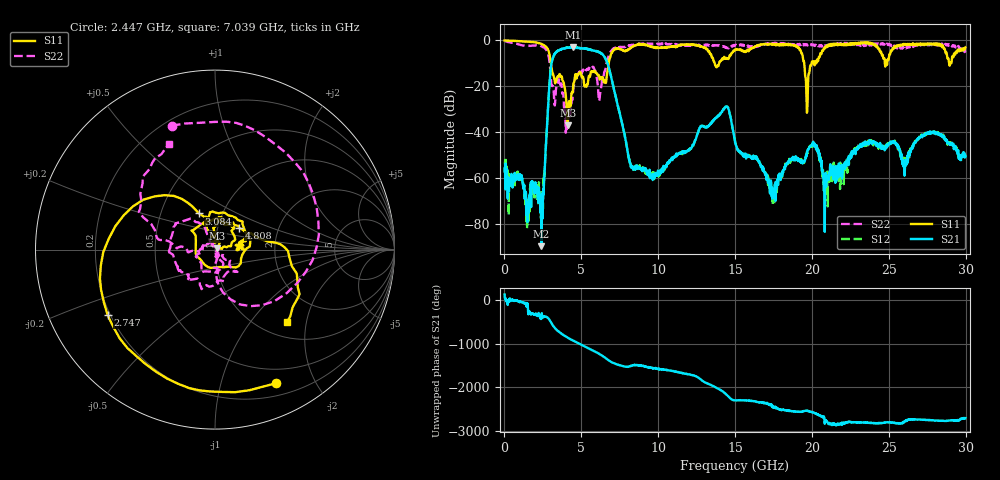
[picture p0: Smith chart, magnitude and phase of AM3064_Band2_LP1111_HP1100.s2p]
# Hz S DB R 50.0
!freq dBS11 angS11 dBS21 angS21 dBS12 angS12 dBS22 angS22
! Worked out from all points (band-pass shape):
!   1600 points, 10 MHz to 29.98 GHz, reference 50 ohm
!   highest |S21| = -3.01 dB at 4.49 GHz (marker M1); lowest = -89.6 dB at 2.409 GHz (marker M2)
!   |S21| within 3 dB of the highest: 3.262 GHz to 6.352 GHz (3.09 GHz wide, 64.3 % of centre)
!   lowest |S11| = -37.1 dB at 4.115 GHz (marker M3), VSWR 1.03, Z = 51.3 + j0.65 ohm
!   |S11| at or under -10 dB: 3.021 GHz to 6.785 GHz (3.764 GHz wide, 76.8 % of centre); 13.68 GHz to 13.96 GHz (280.4 MHz wide, 2.03 % of centre); 19.5 GHz to 19.97 GHz (476.4 MHz wide, 2.41 % of centre)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
!   |S22| runs from -40.2 to -0.1 dB; largest |S21 - S12| = 0.017
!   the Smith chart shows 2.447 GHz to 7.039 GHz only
!   S11 on the Smith chart (normalised r, x): 2.447 GHz: 0.33, -1.51; 2.747 GHz: 0.19, -0.27; 3.084 GHz: 0.78, +0.33; 4.808 GHz: 1.26, +0.32; 7.039 GHz: 1.30, -1.55
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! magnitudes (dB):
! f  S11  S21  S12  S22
! 10 MHz  -0.1  -55.9  -54.2  -0.1
! 1.491 GHz  -0.6  -79.2  -76.3  -2.5
! 2.409 GHz  -1.6  -89.6  -69.8  -2.5
! 2.447 GHz  -1.7  -66.7  -72.6  -2.7
! 2.747 GHz  -3.1  -39.4  -39.3  -4.5
! 3.084 GHz  -13.1  -9.3  -9.3  -19.8
! 4.115 GHz  -37.1  -3.2  -3.2  -38.1
! 4.49 GHz  -18.6  -3.0  -3.1  -20.4
! 4.808 GHz  -14.9  -3.3  -3.2  -14.7
! 5.015 GHz  -15.6  -3.4  -3.3  -14.0
! 6.214 GHz  -16.9  -5.4  -5.3  -23.7
! 7.039 GHz  -4.9  -18.8  -18.8  -3.8
! 8.257 GHz  -3.0  -54.6  -54.9  -1.9
! 10 GHz  -3.3  -58.4  -58.6  -1.7
! 14.39 GHz  -8.0  -28.9  -28.9  -3.2
! 15 GHz  -4.0  -44.6  -44.1  -2.2
! 17.5 GHz  -1.8  -66.9  -67.0  -1.2
! 19.69 GHz  -31.1  -48.9  -48.4  -2.0
! 19.99 GHz  -9.4  -45.8  -46.2  -1.8
! 20.89 GHz  -2.6  -57.7  -64.8  -2.8
! 25 GHz  -8.1  -45.0  -44.6  -1.6
! 29.98 GHz  -3.1  -50.6  -49.6  -4.4
